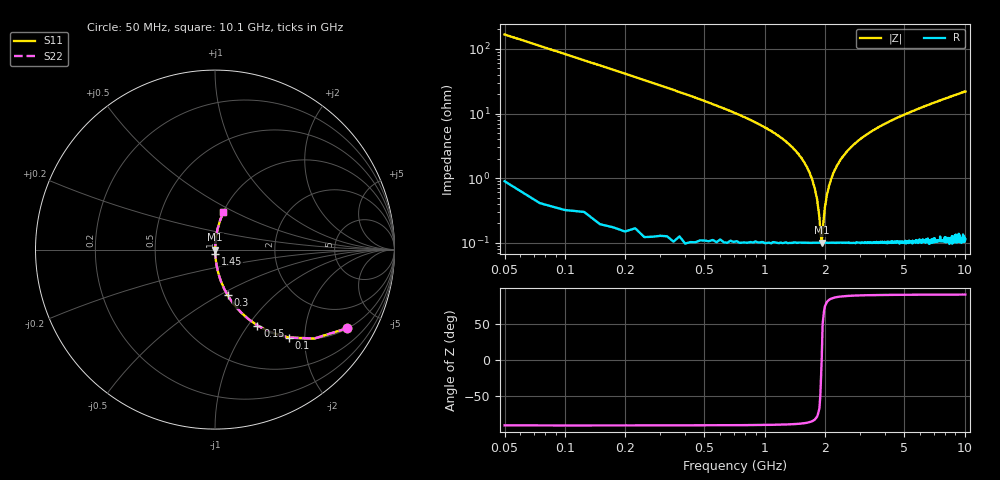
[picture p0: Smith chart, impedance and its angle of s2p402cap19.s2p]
! AVX Thin Film Operation		Date: April 2003
! Description: Accu-P® Series, Thin Film, SMD, RF Capacitor
! Part Number: 0402ZK190FBW
! 50 MHz  -  10.05 GHz
! Serial Measurements
# hz S db R 50
!	S11		S21		S12		S22
!	dB	Phase	dB	Phase	dB	Phase	dB	Phase
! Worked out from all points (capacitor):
!   400 points, 50 MHz to 10.1 GHz, reference 50 ohm
!   read as one part in series: C = 19 pF near 100 MHz
!   lowest |Z| = 100 mohm at 1.93 GHz (marker M1)
!   series resonance near 1.929 GHz, so ESL is about 360 pH
!   S11 on the Smith chart (normalised r, x): 50 MHz: 1.02, -3.34; 100 MHz: 1.01, -1.67; 150 MHz: 1.00, -1.11; 300 MHz: 1.00, -0.55; 1.45 GHz: 1.00, -0.05; 10.1 GHz: 1.00, +0.44
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5e7  -1.35 -30.8  -5.82 58.9  -5.82 58.9  -1.35 -30.8
1e8  -3.88 -50.0  -2.32 39.8  -2.32 39.8  -3.88 -50.0
1.5e8  -6.29 -60.8  -1.18 29.0  -1.18 29.0  -6.29 -60.8
3e8  -11.60 -74.5  -0.32 15.2  -0.32 15.2  -11.60 -74.5
6.75e8  -19.30 -83.2  -0.06 6.2  -0.06 6.2  -19.30 -83.2
1.45e9  -32.10 -86.3  -0.01 1.4  -0.01 1.4  -32.10 -86.3
1.58e9  -35.10 -85.7  -0.01 1.0  -0.01 1.0  -35.10 -85.7
1.73e9  -40.40 -83.5  -0.01 0.5  -0.01 0.5  -40.40 -83.5
1.83e9  -46.50 -77.5  -0.01 0.3  -0.01 0.3  -46.50 -77.5
1.88e9  -52.10 -66.0  -0.01 0.1  -0.01 0.1  -52.10 -66.0
1.9e9  -56.50 -47.9  -0.01 0.1  -0.01 0.1  -56.50 -47.9
1.93e9  -60.00 1.6  -0.01 -0.0  -0.01 -0.0  -60.00 1.6
2e9  -49.10 73.2  -0.01 -0.2  -0.01 -0.2  -49.10 73.2
2.05e9  -45.00 79.4  -0.01 -0.3  -0.01 -0.3  -45.00 79.4
2.15e9  -40.30 83.5  -0.01 -0.6  -0.01 -0.6  -40.30 83.5
2.3e9  -36.10 85.4  -0.01 -0.9  -0.01 -0.9  -36.10 85.4
2.8e9  -29.50 86.4  -0.01 -1.9  -0.01 -1.9  -29.50 86.4
3.4e9  -25.70 85.9  -0.02 -3.0  -0.02 -3.0  -25.70 85.9
5.08e9  -20.20 83.8  -0.05 -5.6  -0.05 -5.6  -20.20 83.8
6.75e9  -17.20 81.6  -0.09 -8.0  -0.09 -8.0  -17.20 81.6
8.43e9  -15.00 79.4  -0.15 -10.2  -0.15 -10.2  -15.00 79.4
1.01e10  -13.40 77.4  -0.21 -12.3  -0.21 -12.3  -13.40 77.4
